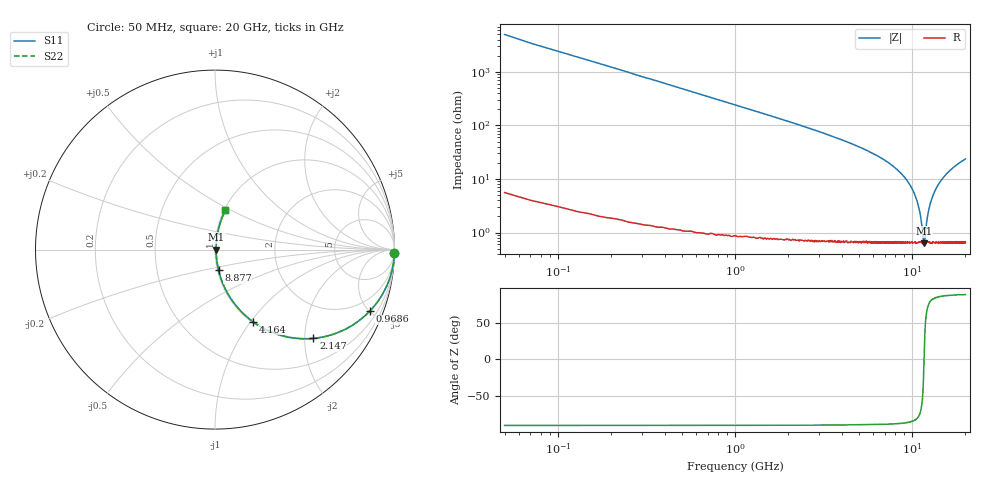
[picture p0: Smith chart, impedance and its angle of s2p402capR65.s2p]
! AVX Thin Film Operation		Date: September 2011
! Description: Accu-P® Series, Thin Film, SMD, RF Capacitor
! Part Number: 04021JR65ZBW/STR
! 50 MHz  -  20 GHz
! Serial Measurements
# MHZ S MA R 50
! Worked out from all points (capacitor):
!   1000 points, 50 MHz to 20 GHz, reference 50 ohm
!   read as one part in series: C = 647 fF near 149.8 MHz
!   lowest |Z| = 627 mohm at 11.69 GHz (marker M1)
!   series resonance near 11.68 GHz, so ESL is about 290 pH
!   S11 on the Smith chart (normalised r, x): 50 MHz: -0, -98; 968.6 MHz: 1.02, -5.02; 2.147 GHz: 1.02, -2.20; 4.164 GHz: 1.01, -1.03; 8.877 GHz: 1.01, -0.23; 20 GHz: 1.01, +0.47
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50  1 -1.2  0.02 88.8  0.02 88.8  1 -1.2
209.76  0.996 -4.9  0.085 85.0  0.085 85.0  0.996 -4.9
369.52  0.989 -8.6  0.149 81.3  0.149 81.3  0.989 -8.6
629.129  0.968 -14.4  0.249 75.4  0.249 75.4  0.968 -14.4
968.619  0.928 -21.7  0.37 68.1  0.37 68.1  0.928 -21.7
1487.838  0.849 -31.6  0.524 58.1  0.524 58.1  0.849 -31.6
2146.847  0.738 -42.0  0.67 47.6  0.67 47.6  0.738 -42.0
3384.985  0.55 -56.1  0.83 33.4  0.83 33.4  0.55 -56.1
4163.814  0.454 -62.2  0.885 27.0  0.885 27.0  0.454 -62.2
6700  0.237 -74.8  0.965 13.7  0.965 13.7  0.237 -74.8
8876.727  0.115 -80.2  0.987 6.6  0.987 6.6  0.115 -80.2
10034.99  0.064 -80.6  0.992 3.6  0.992 3.6  0.064 -80.6
10953.6  0.028 -75.0  0.993 1.5  0.993 1.5  0.028 -75.0
11273.12  0.016 -65.8  0.993 0.9  0.993 0.9  0.016 -65.8
11592.64  0.007243 -26.8  0.994 0.2  0.994 0.2  0.007243 -26.8
11692.49  0.00646 2.5  0.994 -0.0  0.994 -0.0  0.00646 2.5
12391.44  0.025 73.8  0.993 -1.4  0.993 -1.4  0.025 73.8
12810.81  0.039 78.3  0.993 -2.2  0.993 -2.2  0.039 78.3
13350  0.056 80.2  0.992 -3.2  0.992 -3.2  0.056 80.2
14687.99  0.096 80.7  0.989 -5.5  0.989 -5.5  0.096 80.7
16684.99  0.15 78.9  0.982 -8.6  0.982 -8.6  0.15 78.9
20000  0.229 75.2  0.967 -13.2  0.967 -13.2  0.229 75.2
